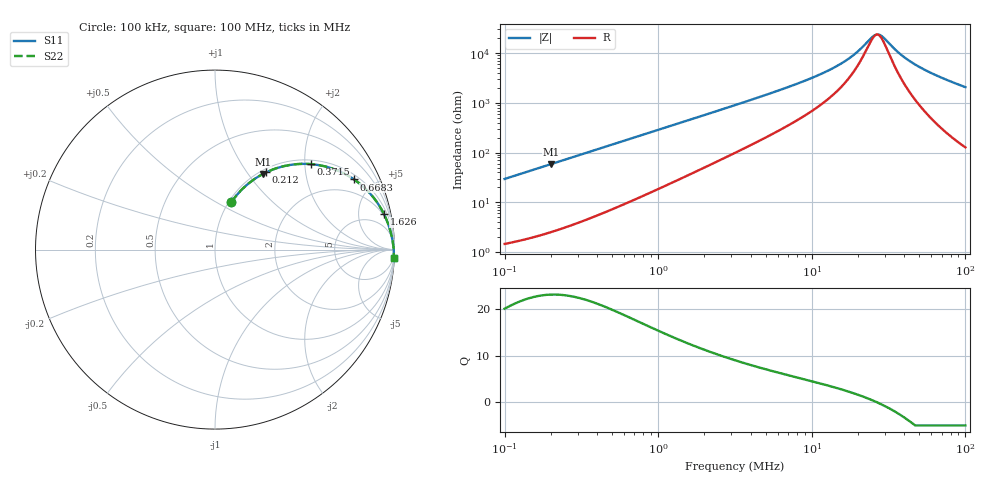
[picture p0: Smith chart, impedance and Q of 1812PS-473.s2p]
# MHz S MA R 50
!Freq  MagS11  AngS11  MagS21  AngS21  MagS12  AngS12  MagS22  AngS22
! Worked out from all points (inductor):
!   801 points, 100 kHz to 100 MHz, reference 50 ohm
!   read as one part in series: L = 46.8 uH near 103.5 kHz
!   highest Q = 23.2 at 201.3 kHz (marker M1), where L = 46.5 uH
!   self-resonance near 26.45 MHz
!   S11 on the Smith chart (normalised r, x): 100 kHz: 1.03, +0.59; 212 kHz: 1.05, +1.24; 371.5 kHz: 1.10, +2.15; 668.3 kHz: 1.21, +3.84; 1.626 MHz: 1.74, +9.22; 100 MHz: 4, -41
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0.1  0.2798 70.9  0.9463 -16.2  0.9463 -16.2  0.2798 70.9
0.1424787  0.3805 65.1  0.9079 -22.3  0.9079 -22.3  0.3805 65.1
0.2012565  0.4982 57.7  0.8459 -29.8  0.8459 -29.8  0.4982 57.7
0.2119581  0.5169 56.4  0.834 -31.1  0.834 -31.1  0.5169 56.4
0.3180534  0.6642 45.9  0.7184 -41.6  0.7184 -41.6  0.6642 45.9
0.3715352  0.7167 41.6  0.6651 -45.7  0.6651 -45.7  0.7167 41.6
0.6683439  0.8677 26.8  0.4514 -60.0  0.4514 -60.0  0.8677 26.8
1.002882  0.9258 18.8  0.3228 -67.5  0.3228 -67.5  0.9258 18.8
1.626485  0.9616 12.0  0.2079 -73.4  0.2079 -73.4  0.9616 12.0
3.162278  0.982 6.2  0.1094 -77.4  0.1094 -77.4  0.982 6.2
6.309573  0.9901 3.0  0.05374 -77.8  0.05374 -77.8  0.9901 3.0
10.05773  0.9928 1.7  0.03121 -75.7  0.03121 -75.7  0.9928 1.7
13.48963  0.9939 1.1  0.0206 -72.3  0.0206 -72.3  0.9939 1.1
16.88496  0.9947 0.7  0.01374 -66.8  0.01374 -66.8  0.9947 0.7
19.72423  0.9951 0.5  0.009521 -58.8  0.009521 -58.8  0.9951 0.5
25.77805  0.9957 0.0  0.004358 -10.1  0.004358 -10.1  0.9957 0.0
28.10283  0.9959 -0.1  0.004418 21.0  0.004418 21.0  0.9959 -0.1
31.71393  0.9961 -0.3  0.006285 51.3  0.006285 51.3  0.9961 -0.3
38.68121  0.9964 -0.6  0.01119 70.7  0.01119 70.7  0.9964 -0.6
48.83711  0.9966 -1.0  0.01813 78.6  0.01813 78.6  0.9966 -1.0
67.22023  0.9966 -1.7  0.02957 82.5  0.02957 82.5  0.9966 -1.7
100  0.9959 -2.8  0.04829 83.7  0.04829 83.7  0.9959 -2.8
